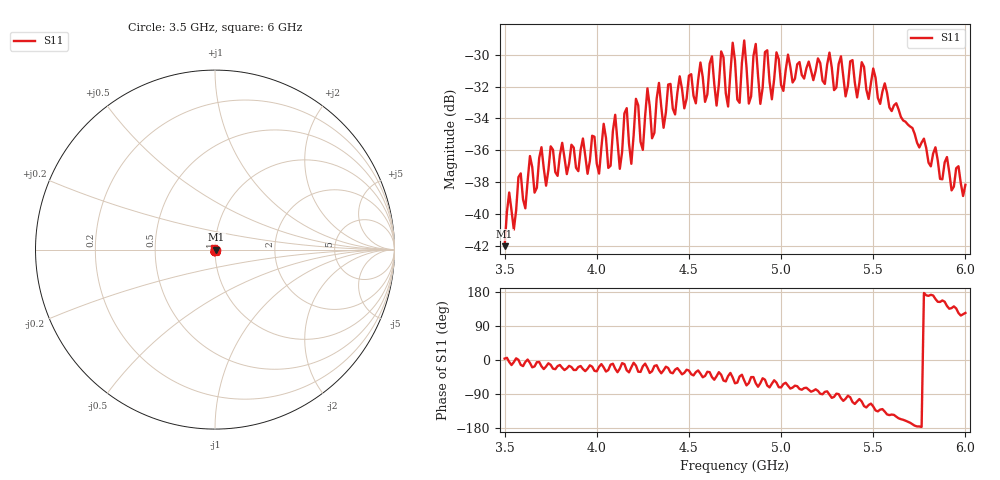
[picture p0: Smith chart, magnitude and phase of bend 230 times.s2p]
!  31/07/2025  13:27:33
! Ref Plane: 0.000 mm
# MHZ S MA R  50
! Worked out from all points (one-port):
!   201 points, 3.5 GHz to 6 GHz, reference 50 ohm
!   lowest |S11| = -42.0 dB at 3.5 GHz (marker M1), VSWR 1.02, Z = 50.8 + j0.0512 ohm
!   |S11| at or under -10 dB: start of sweep to end of sweep
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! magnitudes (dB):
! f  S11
! 3.5 GHz  -42.0
! 3.525 GHz  -38.6
! 3.55 GHz  -41.0
! 3.638 GHz  -36.4
! 3.812 GHz  -35.5
! 4.013 GHz  -37.5
! 4.1 GHz  -33.8
! 4.125 GHz  -37.2
! 4.162 GHz  -33.4
! 4.188 GHz  -36.8
! 4.213 GHz  -32.8
! 4.25 GHz  -36.0
! 4.275 GHz  -32.1
! 4.3 GHz  -35.2
! 4.338 GHz  -31.8
! 4.362 GHz  -34.6
! 4.438 GHz  -32.4
! 4.625 GHz  -30.1
! 4.65 GHz  -33.2
! 4.675 GHz  -29.8
! 4.713 GHz  -33.3
! 4.75 GHz  -30.4
! 4.775 GHz  -33.0
! 4.8 GHz  -29.1
! 5.062 GHz  -31.7
! 5.375 GHz  -30.4
! 5.688 GHz  -34.4
! 6 GHz  -38.2
